[IBIS ver]   4.2
[File name]   tm4c123gh6zrb_157bga_v0p0.ibs
[File Rev]   v0p0
[Date]   Sep 20, 2013
[Source]   simulation
[Notes]   IBIS models for 157BGA package with updated GPIO models
[Disclaimer] Please be aware that in the absence of a written agreement,
   Texas Instruments (TI) assumes no liability for: 1) the
   accuracy of the IBIS models provided to your company, 2) the
   proper functioning of these IBIS models in your design or for
   any resulting applications, or; 3) infringement of patents,
   copyrights, or intellectual property rights resulting from
   your use of these IBIS models. TI provides IBIS models as a
   service to our customers and therefore reserves the right to
   limit distribution of the IBIS models.
   This preliminary model does not contain all of the possible pad
   models for each of the pad types.  The most commonly used modes
   have been provided and the next update will include all of the
   pad model combinations.
   The only missing model that needs to be highlighted is the
   model for the USB D+ and D- GPIOs.  Currently only the USB
   functionality is provided on the D+ and D- pins.  Customers
   needing to model the PGIOs associated with these pins should
   check for a newer model.
[Copyright]   Property of Texas Instruments Incorporated. Unauthorized
   reproduction and/or distribution is strictly prohibited. This
   product is protected under copyright law and trade secret law
   as an unpublished work. Copyright (C) 2013, Texas Instruments
   Incorporated, all rights reserved. These commodities are under
   the U.S. Government distribution license control. As such,
   they are not to be re-exported without the prior approval of
   the U.S. Department of Commerce.
|   Component TM4C123GH6ZRB
[Component]   TM4C123GH6ZRB
[Manufacturer]   Texas Instruments Inc.
[Package]
| 157-pin BGA
| variable   typ   min   max
R_Pkg   1.41E-01   6.35E-02   2.46E-01
L_pkg   1.99E-09   8.11E-10   3.53E-09
C_pkg   5.11E-13   3.53E-13   9.29E-13
[Pin]   signal_name   model_name   R_pin   L_pin   C_pin
A1   GND   GND
A2   NC   NC
A3   PD6   GPIO8P_5V   1.54E-01   2.31E-09   3.98E-13
A4   PD4   GPIO8P_5V   1.44E-01   2.17E-09   3.96E-13
A5   PE4   GPIO8P_5V   2.25E-01   3.09E-09   4.79E-13
A6   PB5   GPIO8P_5V   2.20E-01   2.99E-09   4.78E-13
A7   PE6   GPIO8P_5V   2.25E-01   3.05E-09   4.89E-13
A8   PN0   GPIO8P_5V   2.38E-01   3.27E-09   4.77E-13
A9   PJ2   GPIO8P_5V   1.35E-01   2.14E-09   4.29E-13
A10   PC1_TMS_SWDIO  GPIO8P_5V   1.46E-01   2.22E-09   3.91E-13
A11   PC3_TDO_SWO   GPIO8P_5V   1.57E-01   2.41E-09   3.67E-13
A12   PK7   GPIO8P_5V   1.80E-01   2.78E-09   5.50E-13
A13   PL2   GPIO8P_5V   1.89E-01   3.01E-09   4.79E-13
B1   PD1   GPIO8P_5V   1.61E-01   2.44E-09   4.35E-13
B2   PD0   GPIO8P_5V   1.53E-01   2.29E-09   4.97E-13
B3   PD7   GPIO8P_5V   1.52E-01   2.04E-09   4.69E-13
B4   PD5   GPIO8P_5V   1.40E-01   1.96E-09   4.34E-13
B5   PE5   GPIO8P_5V   2.25E-01   3.01E-09   5.12E-13
B6   PB4   GPIO8P_5V   2.27E-01   3.12E-09   5.37E-13
B7   PE7   GPIO8P_5V   2.30E-01   3.02E-09   5.35E-13
B8   PN1   GPIO8P_5V   2.46E-01   3.49E-09   5.30E-13
B9   PJ1   GPIO8P_5V   1.38E-01   1.87E-09   4.80E-13
B10   PC2_TDI   GPIO8P_5V   1.40E-01   1.96E-09   4.06E-13
B11   PK4   GPIO8P_5V   1.47E-01   2.11E-09   4.13E-13
B12   PK5   GPIO8P_5V   1.47E-01   2.25E-09   4.33E-13
B13   PL3   GPIO8P_5V   1.68E-01   2.66E-09   3.99E-13
C1   PD3   GPIO8P_5V   1.44E-01   2.18E-09   4.20E-13
C2   PD2   GPIO8P_5V   1.47E-01   2.17E-09   4.67E-13
C3   GNDA   GND
C4   PJ7   GPIO8P_5V   1.37E-01   1.86E-09   6.07E-13
C5   PJ5   GPIO8P_5V   1.59E-01   2.05E-09   6.32E-13
C6   PJ6   GPIO8P_5V   8.47E-02   1.09E-09   5.03E-13
C7   GND   GND
C8   PJ3   GPIO8P_5V   8.96E-02   1.15E-09   5.14E-13
C9   PJ0   GPIO8P_5V   9.46E-02   1.20E-09   5.03E-13
C10   PC0_TCK_SWCLK  GPIO8P_5V   1.83E-01   2.40E-09   5.56E-13
C11   PK6   GPIO8P_5V   1.10E-01   1.48E-09   5.59E-13
C12   PL1   GPIO8P_5V   1.07E-01   1.57E-09   5.57E-13
C13   PL5   GPIO8P_5V   1.50E-01   2.28E-09   3.56E-13
D1   VREFAM   NC
D2   VREFAP   NC
D3   VDDA   POWER
D4   PQ0   GPIO8P_5V   1.25E-01   1.54E-09   8.25E-13
D5   PJ4   GPIO8P_5V   1.63E-01   1.96E-09   6.41E-13
D6   VDDC   POWER
D7   VDD   POWER
D8   PP6   GPIO8P_5V   8.02E-02   9.34E-10   5.41E-13
D9   GND   GND
D10   PN3   GPIO8P_5V   2.10E-01   2.67E-09   6.27E-13
D11   PL0   GPIO8P_5V   7.81E-02   9.94E-10   5.90E-13
D12   PL4   GPIO8P_5V   9.38E-02   1.17E-09   3.84E-13
D13   PB3_I2C0SDA   GPIO8P_5V   1.32E-01   2.02E-09   3.52E-13
E1   PE2   GPIO8P_5V   1.41E-01   2.08E-09   3.71E-13
E2   PE3   GPIO8P_5V   1.35E-01   1.95E-09   4.42E-13
E3   GNDA   GND
E4   PQ1   GPIO8P_5V   1.23E-01   1.50E-09   9.28E-13
E5   GND   GND
E6   VDD   POWER
E8   VDD   POWER
E9   VDD   POWER
E10   PB2_I2C0SCL   GPIO8P_5V   1.37E-01   1.74E-09   5.69E-13
E11   PB1_USB0VBUS   GPIO8P_5V   1.69E-01   2.24E-09   5.11E-13
E12   PL6   USB_PHY_DP   1.21E-01   1.71E-09   4.69E-13
E13   PL7   USB_PHY_DM   1.29E-01   1.95E-09   3.99E-13
F1   PE0   GPIO8P_5V   1.20E-01   1.84E-09   4.16E-13
F2   PE1   GPIO8P_5V   1.18E-01   1.64E-09   4.62E-13
F3   PB7   GPIO8P_5V   9.42E-02   1.15E-09   5.22E-13
F4   PB6   GPIO8P_5V   8.46E-02   9.57E-10   4.55E-13
F5   PQ2   GPIO8P_5V   1.67E-01   1.93E-09   6.55E-13
F9   GND   GND
F10   VDD   POWER
F11   PB0_USB0ID   GPIO8P_5V   6.89E-02   8.54E-10   4.51E-13
F12   PM1   GPIO8P_5V   2.15E-01   3.05E-09   6.42E-13
F13   PM0   GPIO8P_5V   1.80E-01   2.61E-09   4.04E-13
G1   PK1   GPIO8P_5V   1.23E-01   1.83E-09   4.14E-13
G2   PK0   GPIO8P_5V   1.26E-01   1.64E-09   4.47E-13
G3   PN2   GPIO8P_5V   6.35E-02   8.10E-10   4.18E-13
G4   PH7   GPIO8P_5V   2.02E-01   2.67E-09   6.16E-13
G10   RST_n   RST_WAKE_INPUT  1.15E-01   1.38E-09   5.79E-13
G11   PM2   GPIO8P_5V   7.84E-02   9.67E-10   4.99E-13
G12   OSC0   NC
G13   OSC1   NC
H1   PK2   GPIO8P_5V   1.23E-01   1.84E-09   3.98E-13
H2   PK3   GPIO8P_5V   1.22E-01   1.71E-09   4.38E-13
H3   PH6   GPIO8P_5V   7.92E-02   9.77E-10   5.00E-13
H4   PH5   GPIO8P_5V   1.22E-01   1.50E-09   5.50E-13
H5   GND   GND
H9   GND   GND
H10   PM3   GPIO8P_5V   1.14E-01   1.42E-09   5.37E-13
H11   PM6   GPIO8P_5V   8.77E-02   1.07E-09   5.09E-13
H12   PM5   GPIO8P_5V   1.19E-01   1.64E-09   4.70E-13
H13   PM4   GPIO8P_5V   1.56E-01   2.30E-09   4.13E-13
J1   VDDC   POWER
J2   PH3   GPIO8P_5V   1.15E-01   1.57E-09   4.74E-13
J3   PH4   GPIO8P_5V   7.96E-02   9.24E-10   7.24E-13
J4   PH2   GPIO8P_5V   1.28E-01   1.61E-09   6.41E-13
J5   GND   GND
J6   VDDC   POWER
J7   VDD   POWER
J8   GND   GND
J9   VDD   POWER
J10   VDD   POWER
J11   GND   GND
J12   PP3   GPIO8P_5V   1.13E-01   1.60E-09   7.80E-13
J13   PP4   GPIO8P_5V   1.80E-01   2.57E-09   6.31E-13
K1   PC6   GPIO8P_5V   1.41E-01   2.15E-09   4.30E-13
K2   PC7   GPIO8P_5V   1.37E-01   1.92E-09   4.69E-13
K3   PH0   GPIO8P_5V   9.56E-02   1.25E-09   6.50E-13
K4   PH1   GPIO8P_5V   1.30E-01   1.57E-09   9.25E-13
K5   PQ5   GPIO8P_5V   1.40E-01   1.82E-09   6.33E-13
K6   PP7   GPIO8P_5V   8.10E-02   9.64E-10   6.85E-13
K7   PG4   GPIO8P_5V   1.33E-01   1.66E-09   5.46E-13
K8   PG1   GPIO8P_5V   9.70E-02   1.12E-09   5.83E-13
K9   PF5   GPIO8P_5V   1.32E-01   1.64E-09   5.54E-13
K10   PF3   GPIO8P_5V   1.55E-01   2.23E-09   6.24E-13
K11   GNDX   GND
K12   VBAT   POWER
K13   VDDC   POWER
L1   PC5   GPIO8P_5V   1.44E-01   2.19E-09   4.01E-13
L2   PC4   GPIO8P_5V   1.50E-01   2.12E-09   4.22E-13
L3   PA0_U0Rx   GPIO8P_5V   7.92E-02   1.11E-09   4.75E-13
L4   PA4_SSI0Rx   GPIO8P_5V   9.73E-02   1.25E-09   7.85E-13
L5   PP5   GPIO8P_5V   9.85E-02   1.27E-09   5.24E-13
L6   PQ7   GPIO8P_5V   9.55E-02   1.11E-09   4.83E-13
L7   PG5   GPIO8P_5V   9.45E-02   1.19E-09   5.24E-13
L8   PG0   GPIO8P_5V   1.03E-01   1.29E-09   5.30E-13
L9   PF4   GPIO8P_5V   9.76E-02   1.24E-09   5.17E-13
L10   PF2   GPIO8P_5V   1.12E-01   1.48E-09   5.40E-13
L11   PN4   GPIO8P_5V   1.85E-01   2.54E-09   5.53E-13
L12   PP1   GPIO8P_5V   1.75E-01   2.61E-09   6.37E-13
L13   PM7   GPIO8P_5V   2.19E-01   3.53E-09   4.61E-13
M1   PA1_U0Tx   GPIO8P_5V   1.67E-01   2.56E-09   4.85E-13
M2   PA2_SSI0Clk   GPIO8P_5V   1.42E-01   2.22E-09   4.80E-13
M3   PA3_SSI0Fss   GPIO8P_5V   1.21E-01   1.77E-09   4.89E-13
M4   PA6   GPIO8P_5V   1.11E-01   1.61E-09   6.39E-13
M5   PP2   GPIO8P_5V   1.28E-01   1.78E-09   5.50E-13
M6   PQ6   GPIO8P_5V   1.30E-01   1.79E-09   4.84E-13
M7   PG3   GPIO8P_5V   1.33E-01   1.85E-09   4.75E-13
M8   PF7   GPIO8P_5V   1.11E-01   1.60E-09   4.42E-13
M9   PF0   GPIO8P_5V   1.29E-01   1.80E-09   4.92E-13
M10   XOSC0   NC
M11   PN7   GPIO8P_5V   1.74E-01   2.48E-09   4.31E-13
M12   HIB_n   HIB_OUTPUT   1.51E-01   2.29E-09   5.98E-13
M13   PP0   GPIO8P_5V   2.14E-01   3.36E-09   5.50E-13
N1   PA5_SSI0Tx   GPIO8P_5V   2.02E-01   3.22E-09   5.67E-13
N2   PA7   GPIO8P_5V   2.02E-01   3.19E-09   5.24E-13
N3   PG7   GPIO8P_5V   1.74E-01   2.66E-09   5.15E-13
N4   PG6   GPIO8P_5V   1.60E-01   2.51E-09   4.90E-13
N5   PQ3   GPIO8P_5V   1.33E-01   2.07E-09   4.50E-13
N6   PQ4   GPIO8P_5V   1.58E-01   2.37E-09   4.09E-13
N7   PG2   GPIO8P_5V   1.37E-01   2.12E-09   3.88E-13
N8   PF6   GPIO8P_5V   1.38E-01   2.12E-09   3.69E-13
N9   PF1   GPIO8P_5V   1.68E-01   2.48E-09   4.15E-13
N10   XOSC1   NC
N11   PN6   GPIO8P_5V   1.48E-01   2.29E-09   3.57E-13
N12   PN5   GPIO8P_5V   1.68E-01   2.59E-09   3.97E-13
N13   WAKE_n   RST_WAKE_INPUT  1.82E-01   2.84E-09   4.68E-13
[Model Selector] GPIO8P_5V
GPIO8P_5V_I/O_2   2mA Output Buffer
GPIO8P_5V_I/O_4   4mA Output Buffer
GPIO8P_5V_I/O_8S   8mA Output Buffer with Slew Rate Control
GPIO8P_5V_I/O_8   8mA Output Buffer
GPIO8P_5V_I_WPU_2   2mA Input with Pull-Up
GPIO8P_5V_I_WPD_2   2mA Input with Pull-Down
GPIO8P_5V_I/O_OD_2   2mA Output Buffer with Open Drain
GPIO8P_5V_I/O_OD_4   4mA Output Buffer with Open Drain
GPIO8P_5V_I/O_OD_8S   8mA Output Buffer with Open Drain and Slew Rate Control
GPIO8P_5V_I/O_OD_8   8mA Output Buffer with Open Drain
[Model Selector] RST_WAKE_INPUT
RST_WAKE_IN   Input Model for the WAKE_n Pin
[Model Selector] HIB_OUTPUT
HIBERNATE_OUTPUT   Output Buffer for the HIB_n Pin
[Model Selector] USB_PHY_DP
fsdp_tx   Full Speed transmitter--12Mbps
lsdp_50pf_tx   Low speed transmitter--1.5Mbps driving 50pF cap load
lsdp_200pf_tx   Low speed transmitter--1.5Mbps driving 200pF cap load
lsdp_400pf_tx   Low speed transmitter--1.5Mbps driving 400pF cap load
lsdp_600pf_tx   Low speed transmitter--1.5Mbps driving 600pF cap load
fsdp_rx   Recieve mode--Open circuit during fs/ls recieve mode
[Model Selector] USB_PHY_DM
fsdm_tx   Full Speed transmitter--12Mbps
lsdm_50pf_tx   Low speed transmitter--1.5Mbps driving 50pF cap load
lsdm_200pf_tx   Low speed transmitter--1.5Mbps driving 200pF cap load
lsdm_400pf_tx   Low speed transmitter--1.5Mbps driving 400pF cap load
lsdm_600pf_tx 	 Low speed transmitter--1.5Mbps driving 600pF cap load
fsdm_rx   Recieve mode--Open circuit during fs/ls recieve mode
| Models and submodels in the file (24): GPIO8P_5V_I/O_2 (I/O), GPIO8P_5V_I/O_4 (I/O), GPIO8P_5V_I/O_8S (I/O), GPIO8P_5V_I/O_8 (I/O), GPIO8P_5V_I_WPU_2 (Input), GPIO8P_5V_I_WPD_2 (Input), GPIO8P_5V_I/O_OD_2 (I/O_open_drain), GPIO8P_5V_I/O_OD_4 (I/O_open_drain), GPIO8P_5V_I/O_OD_8S (I/O_open_drain), GPIO8P_5V_I/O_OD_8 (I/O_open_drain), RST_WAKE_IN (Input), HIBERNATE_OUTPUT (Output), fsdp_tx (3-state), lsdp_50pf_tx (3-state), lsdp_200pf_tx (3-state), lsdp_400pf_tx (3-state), lsdp_600pf_tx (3-state), fsdp_rx (Input), fsdm_tx (3-state), lsdm_50pf_tx (3-state), lsdm_200pf_tx (3-state), lsdm_400pf_tx (3-state), lsdm_600pf_tx (3-state), fsdm_rx (Input)
